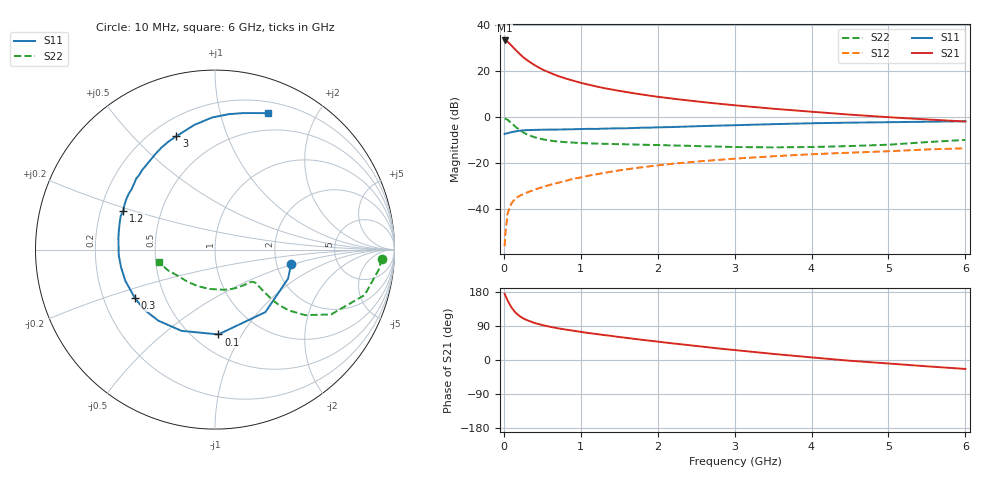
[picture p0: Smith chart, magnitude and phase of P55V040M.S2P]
! SIEMENS Small Signal Semiconductors
! BFP183
! Si NPN RF Bipolar Junction Transistor in SOT143
! VCE = 5 V  IC = 40 mA
! Common Emitter S-Parameters:  March  1996
# GHz  S  MA  R  50
!  f  S11  S21  S12  S22
! GHz  MAG  ANG  MAG  ANG  MAG  ANG  MAG  ANG
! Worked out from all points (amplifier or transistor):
!   36 points, 10 MHz to 6 GHz, reference 50 ohm
!   highest |S21| = 33.2 dB at 10 MHz (marker M1)
!   |S21| within 3 dB of that: start of sweep to 121.3 MHz
!   unconditionally stable (mu >= 1): 564.7 MHz to 5.814 GHz
!   at 250 MHz: K = 0.65, MSG = 29.7 dB, |S12| = -33.4 dB
!   at 1.4 GHz: K = 1.19, MAG = 15.1 dB, |S12| = -23.6 dB
!   at 6 GHz: K = 0.98, MSG = 5.8 dB, |S12| = -13.5 dB
!   S11 on the Smith chart (normalised r, x): 10 MHz: 2.41, -0.46; 100 MHz: 0.65, -0.80; 300 MHz: 0.34, -0.25; 1.2 GHz: 0.30, +0.19; 3 GHz: 0.30, +0.67; 6 GHz: 0.31, +1.41
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0.01  0.4317 -10.4  45.81 174.8  0.0016 81.0  0.9299 -3.1
0.02  0.4379 -21.7  45.55 170.4  0.003 83.5  0.9204 -6.8
0.05  0.4474 -51.1  42.77 156.4  0.0083 74.0  0.8712 -16.9
0.1  0.4729 -87.7  35.32 138.4  0.0136 60.5  0.7406 -29.2
0.15  0.4897 -112.4  28.91 125.5  0.0173 54.8  0.6212 -36.0
0.2  0.5064 -128.6  23.87 116.6  0.0195 53.4  0.5331 -39.5
0.25  0.5181 -140.1  20 110.0  0.0213 51.6  0.4695 -40.9
0.3  0.5215 -149.0  17.25 105.3  0.0232 52.0  0.4227 -41.2
0.4  0.5291 -160.9  13.36 97.6  0.0269 53.6  0.3657 -40.8
0.5  0.5328 -169.5  10.78 92.2  0.0304 54.4  0.3314 -40.2
0.6  0.5369 -176.5  9.138 87.7  0.0341 56.6  0.3102 -39.7
0.7  0.5377 178.1  7.819 83.8  0.0376 57.5  0.2963 -39.4
0.8  0.5422 172.9  6.914 80.4  0.0414 58.0  0.2873 -39.6
1.1  0.5578 160.3  5.051 71.2  0.0537 58.6  0.2698 -41.8
1.2  0.5551 156.9  4.623 68.7  0.0576 58.0  0.2671 -43.0
1.7  0.582 140.7  3.265 55.7  0.0782 55.5  0.2551 -51.1
2.2  0.6103 127.5  2.51 43.7  0.0978 51.7  0.243 -61.4
3  0.6673 108.8  1.807 26.3  0.1258 44.0  0.2248 -82.5
3.5  0.7042 99.4  1.521 16.1  0.1419 39.4  0.2213 -97.9
4.5  0.7587 84.1  1.132 -2.0  0.1698 29.8  0.2361 -131.0
5.5  0.7942 73.3  0.891 -16.7  0.1994 21.6  0.2874 -156.5
6  0.8154 68.8  0.803 -23.6  0.2113 16.9  0.321 -167.4
